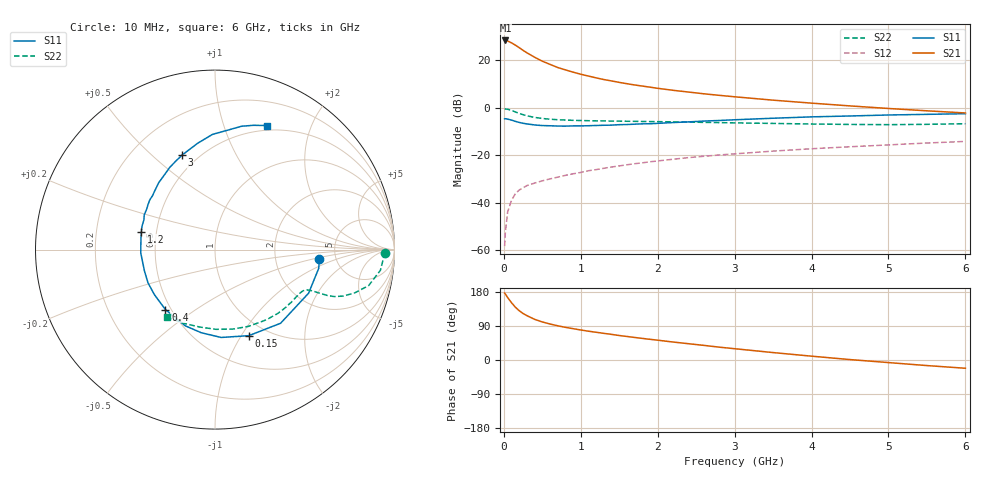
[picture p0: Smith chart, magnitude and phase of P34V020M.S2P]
! SIEMENS Small Signal Semiconductors
! BFP181
! Si NPN RF Bipolar Junction Transistor in SOT143
! VCE = 4 V  IC = 20 mA
! Common Emitter S-Parameters:  March  1996
# GHz  S  MA  R  50
!  f  S11  S21  S12  S22
! GHz  MAG  ANG  MAG  ANG  MAG  ANG  MAG  ANG
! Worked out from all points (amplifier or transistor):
!   36 points, 10 MHz to 6 GHz, reference 50 ohm
!   highest |S21| = 28.4 dB at 20 MHz (marker M1)
!   |S21| within 3 dB of that: start of sweep to 197.8 MHz
!   unconditionally stable (mu >= 1): start of sweep to 12.34 MHz; 595.8 MHz to end of sweep
!   at 250 MHz: K = 0.57, MSG = 29.0 dB, |S12| = -33.8 dB
!   at 1.4 GHz: K = 1.31, MAG = 14.8 dB, |S12| = -25.0 dB
!   at 6 GHz: K = 1.05, MAG = 4.6 dB, |S12| = -14.2 dB
!   S11 on the Smith chart (normalised r, x): 10 MHz: 3.70, -0.59; 150 MHz: 0.83, -1.08; 400 MHz: 0.47, -0.38; 1.2 GHz: 0.41, +0.10; 3 GHz: 0.41, +0.63; 6 GHz: 0.45, +1.40
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0.01  0.5839 -5.2  26.26 176.6  0.0012 73.1  0.9461 -1.0
0.02  0.5873 -10.2  26.29 174.0  0.0024 87.2  0.9414 -2.6
0.05  0.5754 -24.9  25.63 164.7  0.0064 81.7  0.9284 -7.2
0.1  0.5495 -48.3  23.36 151.1  0.0111 66.6  0.879 -13.2
0.15  0.5151 -68.6  20.92 139.3  0.0154 62.3  0.8151 -17.2
0.2  0.4907 -86.0  18.51 130.0  0.0184 59.4  0.7608 -19.9
0.25  0.4694 -99.4  16.24 122.7  0.0204 56.5  0.7139 -21.5
0.3  0.4558 -111.3  14.43 117.0  0.0228 54.5  0.6771 -22.2
0.4  0.4334 -129.6  11.63 107.3  0.0257 53.3  0.6246 -22.7
0.5  0.4207 -143.6  9.601 100.4  0.0287 52.8  0.5935 -22.9
0.6  0.4166 -153.7  8.221 95.0  0.0315 53.7  0.5731 -23.3
0.7  0.4107 -163.2  7.067 90.3  0.0343 54.5  0.5588 -23.7
0.9  0.4139 -177.3  5.637 82.7  0.0404 55.7  0.5425 -25.0
1.1  0.4174 171.1  4.658 76.0  0.0469 56.1  0.5326 -26.9
1.2  0.4223 166.2  4.269 73.2  0.0495 56.1  0.5291 -28.0
1.7  0.4501 145.9  3.023 59.5  0.0659 55.6  0.5168 -34.6
2.2  0.4874 130.0  2.333 47.4  0.0819 53.2  0.5037 -42.3
3  0.5573 109.3  1.703 29.8  0.1065 47.9  0.4794 -56.3
3.5  0.6007 99.2  1.445 19.6  0.1216 44.3  0.4667 -66.4
4.5  0.6698 83.8  1.093 1.1  0.1502 36.3  0.4442 -89.3
5.5  0.7254 72.7  0.861 -14.7  0.1803 28.6  0.4466 -113.3
6  0.7487 67.4  0.776 -21.8  0.1947 24.0  0.4601 -125.2
